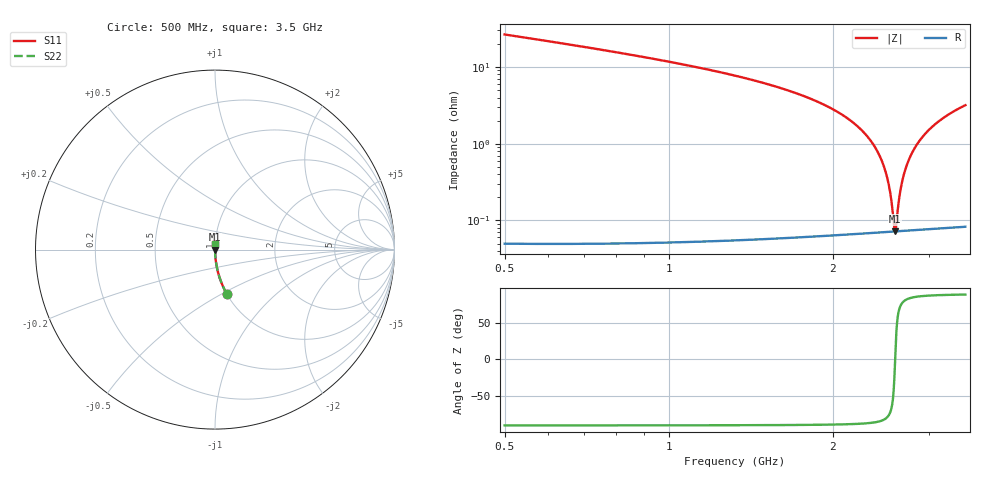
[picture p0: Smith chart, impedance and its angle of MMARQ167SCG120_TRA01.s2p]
! MMARQ167SCG120_TRA01  S-PARAMETER MODEL  ( General Type )
! Model Generated by TAIYO YUDEN Corporation (http://www.ty-top.com)
! Version 1.0
! TAIYO YUDEN Control No. 150305
! Copyright(c) 2015 TAIYO YUDEN CO.,LTD. All Rights Reserved.
! Product Description (link to TY-COMPAS)
! https://ds.yuden.co.jp/TYCOMPAS/or/detail?pn=MMARQ167SCG120JTRA01&u=M
! Products Name : Multilayer Ceramic Capacitors
! Characteristics :
!  Capacitance : 12 pF , Rated Voltage : 250V , TCC : CG / C0G
!  Case Size : 1.6 x 0.8 / 0.063 x 0.031 [mm/inch] , Thickness : 0.7 / 0.028 [mm/inch]
!  (Conditions: Temperature = 25 degC , DC Bias Current/Voltage = 0A / 0V)
! External Node Assignments :
!  1  o---| |---o  2
! GND o---------o GND
! Frequency Range : 500MHz  -  3.5GHz  [ 401 STEP ]
# MHz S RI R 50
! Freq[MHz].  S11 Real  S11 Imag  S21 Real  S21 Imag  S12 Real  S12 Imag  S22 Real  S22 Imag
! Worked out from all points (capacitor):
!   401 points, 500 MHz to 3.5 GHz, reference 50 ohm
!   read as one part in series: C = 11.6 pF near 515 MHz
!   lowest |Z| = 72.1 mohm at 2.6 GHz (marker M1)
!   series resonance near 2.601 GHz, so ESL is about 320 pH
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500  0.0661 -0.2476  0.9339 0.2476  0.9339 0.2476  0.0661 -0.2476
725  0.0302 -0.1698  0.9698 0.1698  0.9698 0.1698  0.0302 -0.1698
1002.5  0.014 -0.1152  0.986 0.1152  0.986 0.1152  0.014 -0.1152
1505  0.00425 -0.0605  0.9957 0.0605  0.9957 0.0605  0.00425 -0.0605
2000  0.00143 -0.0281  0.9986 0.0281  0.9986 0.0281  0.00143 -0.0281
2180  0.00101 -0.0187  0.999 0.0187  0.999 0.0187  0.00101 -0.0187
2322.5  0.000825 -0.012  0.9992 0.012  0.9992 0.012  0.000825 -0.012
2427.5  0.000749 -0.0073  0.9993 0.0073  0.9993 0.0073  0.000749 -0.0073
2502.5  0.000722 -0.00409  0.9993 0.00409  0.9993 0.00409  0.000722 -0.00409
2547.5  0.000716 -0.00221  0.9993 0.00221  0.9993 0.00221  0.000716 -0.00221
2585  0.000717 -0.000663  0.9993 0.000663  0.9993 0.000663  0.000717 -0.000663
2600  0.000718 -5.3e-05  0.9993 5.3e-05  0.9993 5.3e-05  0.000718 -5.3e-05
2615  0.00072 0.000554  0.9993 -0.000554  0.9993 -0.000554  0.00072 0.000554
2645  0.000727 0.00176  0.9993 -0.00176  0.9993 -0.00176  0.000727 0.00176
2667.5  0.000734 0.00265  0.9993 -0.00265  0.9993 -0.00265  0.000734 0.00265
2697.5  0.000745 0.00383  0.9993 -0.00383  0.9993 -0.00383  0.000745 0.00383
2735  0.000764 0.00529  0.9992 -0.00529  0.9992 -0.00529  0.000764 0.00529
2787.5  0.000796 0.0073  0.9992 -0.0073  0.9992 -0.0073  0.000796 0.0073
2847.5  0.000841 0.00955  0.9992 -0.00955  0.9992 -0.00955  0.000841 0.00955
3005  0.001 0.0153  0.999 -0.0153  0.999 -0.0153  0.001 0.0153
3222.5  0.00131 0.0227  0.9987 -0.0227  0.9987 -0.0227  0.00131 0.0227
3500  0.00183 0.0317  0.9982 -0.0317  0.9982 -0.0317  0.00183 0.0317
